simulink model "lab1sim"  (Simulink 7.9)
settings: Solver=ode45  SolverMode=SingleTasking  StartTime=0.0  StopTime=2  FixedStep=0.001  RelTol=1e-3
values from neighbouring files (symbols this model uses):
  C = lC    [initlab1sim.m]
  dDZ = 0.1    [initlab1sim.m]
  dzpos = 0    [initlab1sim.m]
  DZPOS = 0    [initlab1sim.m]
  GAM = lGAM    [initlab1sim.m]
  h = 0.001    [dfa.m]    (also in initlab1sim.m)
  K = lK    [initlab1sim.m]    (also in lqed.m = Phi*Kf+Kv)
  Lc = lLc    (= 1)    [initlab1sim.m]
  Le = lLe    [initlab1sim.m]
  overlap = 0    [fix_opencfg.m]    (also in initlab1sim.m)
  OVERLAP = 2    [initlab1sim.m]
  PHI = lPHI    [initlab1sim.m]
  tl = + 1.3    (= 1.3)    [initlab1sim.m]
  TL = + 1.3    (= 1.3)    [initlab1sim.m]
  tu = - 1.0    (= -1)    [initlab1sim.m]
  TU = - 1.0    (= -1)    [initlab1sim.m]
undefined symbols (not defined in the file or in its folder): DiscIntNeverNeededParam, SimDen, SimNum
libraries: simulink x2, simulink_extras x1

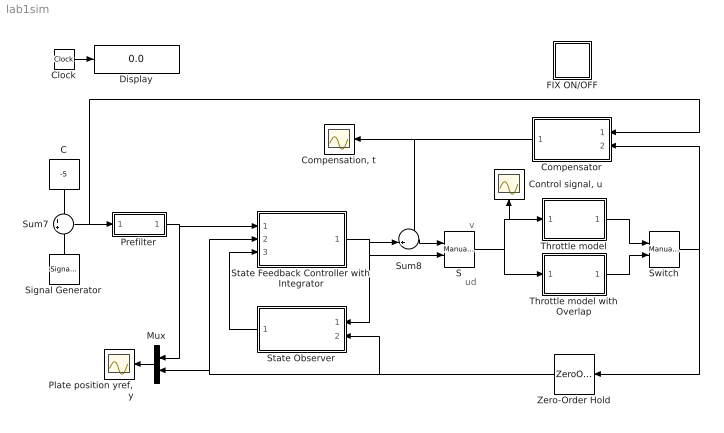
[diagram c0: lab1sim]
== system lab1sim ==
  note: v
  note: ud
  C : Constant  Value=-5
  Clock : Clock
  "Compensation, t" : Scope
  Compensator : Subsystem
  "Control signal, u" : Scope
  Display : Display
  FIX ON/OFF : Subsystem  Description=Fix ON/OFF
  Mux : Mux  Inputs=2
  "Plate position yref, y" : Scope
  Prefilter : Subsystem
  S : simulink/Signal Routing/Manual Switch  sw=0  action=0  varsize=off
  Signal Generator : SignalGenerator  WaveForm=square  Amplitude=5
  State Feedback Controller with Integrator : Subsystem
  State Observer : Subsystem
  Sum7 : Sum
  Sum8 : Sum  Inputs=-+|
  Switch : simulink/Signal Routing/Manual Switch  sw=1  action=0  varsize=off
  Throttle model : Subsystem
  Throttle model with Overlap : Subsystem
  Zero-Order Hold : ZeroOrderHold  SampleTime=h
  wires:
  Signal Generator/1 -> Sum7/2
  Prefilter/1(rfiltered) -> Mux/1, State Feedback Controller with Integrator/1(yr)
  Mux/1 -> "Plate position yref, y"/1
  Zero-Order Hold/1 -> State Observer/2(y), Mux/2, State Feedback Controller with Integrator/2(y)
  State Observer/1(xhat) -> State Feedback Controller with Integrator/3(xhat)
  Sum7/1 -> Prefilter/1(r), Compensator/1(ref.value)
  Switch/1 -> Zero-Order Hold/1, Compensator/2(y)
  Sum8/1 -> S/1
  State Feedback Controller with Integrator/1(ud) -> Sum8/2, S/2, State Observer/1(u)
  Throttle model with Overlap/1(y) -> Switch/2
  Throttle model/1(y) -> Switch/1
  S/1 -> Throttle model/1(u), "Control signal, u"/1, Throttle model with Overlap/1(u)
  Compensator/1(t) -> Sum8/1, "Compensation, t"/1
  Clock/1 -> Display/1
  C/1 -> Sum7/1

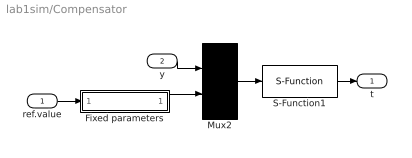
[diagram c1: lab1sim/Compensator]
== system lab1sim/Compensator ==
  ref.value : Inport
  y : Inport  Port=2
  Fixed parameters : Subsystem
  Mux2 : Mux  Inputs=2
  S-Function1 : S-Function  FunctionName=compensator2  Parameters=h overlap/2 -overlap/2  EnableBusSupport=off
  t : Outport
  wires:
  ref.value/1 -> Fixed parameters/1(ref value)
  y/1 -> Mux2/1
  Mux2/1 -> S-Function1/1
  S-Function1/1 -> t/1
  Fixed parameters/1(params) -> Mux2/2

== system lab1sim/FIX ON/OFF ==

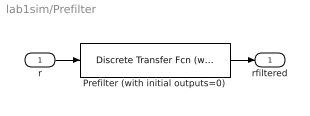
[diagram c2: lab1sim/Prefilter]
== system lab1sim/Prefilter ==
  r : Inport
  Prefilter (with initial outputs=0) : simulink_extras/Additional Discrete/Discrete Transfer Fcn (with initial outputs)  N=[21.3 1 -20.3]  D=[835 -1596 763]  U0=[0]  Y0=0  TS=h
  rfiltered : Outport
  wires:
  Prefilter (with initial outputs=0)/1 -> rfiltered/1
  r/1 -> Prefilter (with initial outputs=0)/1

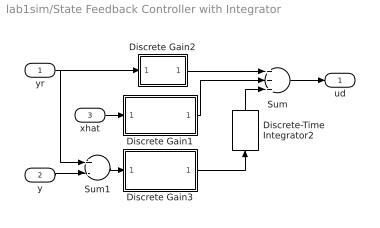
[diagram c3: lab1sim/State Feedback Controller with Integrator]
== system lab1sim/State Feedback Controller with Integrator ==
  yr : Inport
  y : Inport  Port=2
  xhat : Inport  Port=3
  Discrete Gain1 : Subsystem  mask(Discrete Gain){h=h, K=-Le(1:3)}
      mask prompts: h "Sample Time"; K "Gain"
      mask init:
      | s = get_param(gcb,'MaskValueString');
      | s = s(findstr(s,'|')+1:end);
  Discrete Gain2 : Subsystem  mask(Discrete Gain){h=h, K=Lc}
      mask prompts: h "Sample Time"; K "Gain"
      mask init:
      | s = get_param(gcb,'MaskValueString');
      | s = s(findstr(s,'|')+1:end);
  Discrete Gain3 : Subsystem  mask(Discrete Gain){h=h, K=-Le(4)}
      mask prompts: h "Sample Time"; K "Gain"
      mask init:
      | s = get_param(gcb,'MaskValueString');
      | s = s(findstr(s,'|')+1:end);
  Discrete-Time Integrator2 : DiscreteIntegrator  SampleTime=h  ICPrevOutput=DiscIntNeverNeededParam  ICPrevScaledInput=DiscIntNeverNeededParam
  Sum : Sum  Inputs=+++
  Sum1 : Sum  Inputs=+-
  ud : Outport
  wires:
  Discrete Gain1/1(Out1) -> Sum/2
  Discrete-Time Integrator2/1 -> Sum/3
  Sum/1 -> ud/1
  Discrete Gain3/1(Out1) -> Discrete-Time Integrator2/1
  Discrete Gain2/1(Out1) -> Sum/1
  xhat/1 -> Discrete Gain1/1(In1)
  y/1 -> Sum1/2
  yr/1 -> Discrete Gain2/1(In1), Sum1/1
  Sum1/1 -> Discrete Gain3/1(In1)

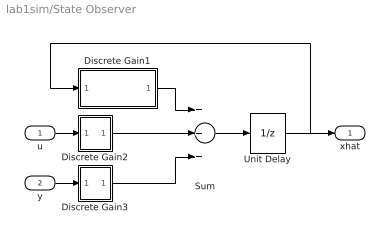
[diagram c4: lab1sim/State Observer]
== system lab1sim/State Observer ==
  u : Inport
  y : Inport  Port=2
  Discrete Gain1 : Subsystem  mask(Discrete Gain){h=h, K=PHI-K*C}
      mask prompts: h "Sample Time"; K "Gain"
      mask init:
      | s = get_param(gcb,'MaskValueString');
      | s = s(findstr(s,'|')+1:end);
  Discrete Gain2 : Subsystem  mask(Discrete Gain){h=h, K=GAM}
      mask prompts: h "Sample Time"; K "Gain"
      mask init:
      | s = get_param(gcb,'MaskValueString');
      | s = s(findstr(s,'|')+1:end);
  Discrete Gain3 : Subsystem  mask(Discrete Gain){h=h, K=K}
      mask prompts: h "Sample Time"; K "Gain"
      mask init:
      | s = get_param(gcb,'MaskValueString');
      | s = s(findstr(s,'|')+1:end);
  Sum : Sum  Inputs=+++
  Unit Delay : UnitDelay  SampleTime=h
  xhat : Outport
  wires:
  Discrete Gain1/1(Out1) -> Sum/1
  Discrete Gain2/1(Out1) -> Sum/2
  Discrete Gain3/1(Out1) -> Sum/3
  Sum/1 -> Unit Delay/1
  Unit Delay/1 -> Discrete Gain1/1(In1), xhat/1
  u/1 -> Discrete Gain2/1(In1)
  y/1 -> Discrete Gain3/1(In1)

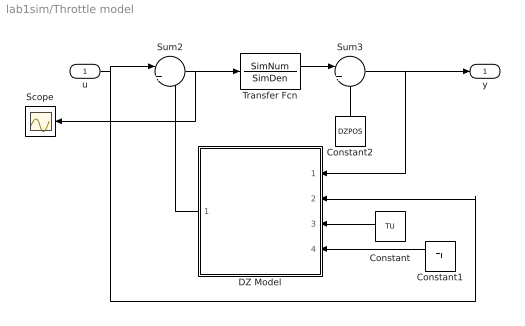
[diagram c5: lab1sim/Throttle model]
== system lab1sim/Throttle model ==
  u : Inport
  Constant : Constant  Value=TU
  Constant1 : Constant  Value=TL
  Constant2 : Constant  Value=DZPOS
  DZ Model : Subsystem
  Scope : Scope
  Sum2 : Sum  Inputs=|++
  Sum3 : Sum  Inputs=|++
  Transfer Fcn : TransferFcn  Numerator=SimNum  Denominator=SimDen
  y : Outport
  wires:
  Sum3/1 -> DZ Model/1(position), y/1
  Constant2/1 -> Sum3/2
  Transfer Fcn/1 -> Sum3/1
  u/1 -> DZ Model/2(torque), Sum2/1
  Constant/1 -> DZ Model/3(TU)
  Constant1/1 -> DZ Model/4(TL)
  Sum2/1 -> Transfer Fcn/1, Scope/1
  DZ Model/1(dz) -> Sum2/2

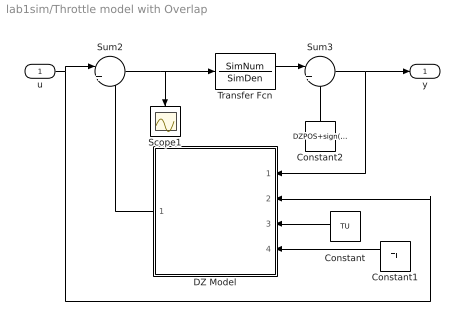
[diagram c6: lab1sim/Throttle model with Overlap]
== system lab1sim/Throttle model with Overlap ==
  u : Inport
  Constant : Constant  Value=TU
  Constant1 : Constant  Value=TL
  Constant2 : Constant  Value=DZPOS+sign(TU+TL)*OVERLAP/2
  DZ Model : Subsystem
  Scope1 : Scope
  Sum2 : Sum  Inputs=|++
  Sum3 : Sum  Inputs=|++
  Transfer Fcn : TransferFcn  Numerator=SimNum  Denominator=SimDen
  y : Outport
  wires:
  Sum3/1 -> DZ Model/1(position), y/1
  Constant2/1 -> Sum3/2
  Transfer Fcn/1 -> Sum3/1
  Sum2/1 -> Scope1/1, Transfer Fcn/1
  Constant1/1 -> DZ Model/4(TL)
  Constant/1 -> DZ Model/3(TU)
  u/1 -> DZ Model/2(torque), Sum2/1
  DZ Model/1(dz) -> Sum2/2

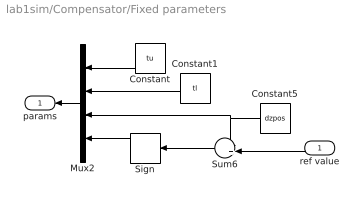
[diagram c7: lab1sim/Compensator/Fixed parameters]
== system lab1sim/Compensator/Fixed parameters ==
  ref value : Inport
  Constant : Constant  Value=tu
  Constant1 : Constant  Value=tl
  Constant5 : Constant  Value=dzpos
  Mux2 : Mux
  Sign : Signum
  Sum6 : Sum  Inputs=-+|
  params : Outport
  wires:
  Sign/1 -> Mux2/4
  Constant/1 -> Mux2/1
  Constant5/1 -> Mux2/3, Sum6/1
  ref value/1 -> Sum6/2
  Sum6/1 -> Sign/1
  Constant1/1 -> Mux2/2
  Mux2/1 -> params/1

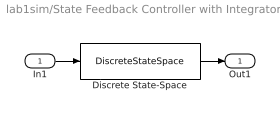
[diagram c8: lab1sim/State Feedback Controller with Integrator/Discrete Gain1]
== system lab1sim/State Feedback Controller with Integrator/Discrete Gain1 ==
  In1 : Inport
  Discrete State-Space : DiscreteStateSpace  A=0  B=zeros(1,size(K,2))  C=zeros(size(K,1),1)  D=K  SampleTime=h
  Out1 : Outport
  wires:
  Discrete State-Space/1 -> Out1/1
  In1/1 -> Discrete State-Space/1

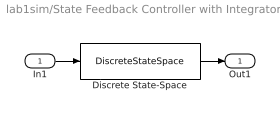
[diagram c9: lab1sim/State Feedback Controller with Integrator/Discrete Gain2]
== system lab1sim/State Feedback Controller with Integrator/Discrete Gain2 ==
  In1 : Inport
  Discrete State-Space : DiscreteStateSpace  A=0  B=zeros(1,size(K,2))  C=zeros(size(K,1),1)  D=K  SampleTime=h
  Out1 : Outport
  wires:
  Discrete State-Space/1 -> Out1/1
  In1/1 -> Discrete State-Space/1

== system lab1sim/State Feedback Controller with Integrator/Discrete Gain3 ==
  In1 : Inport
  Discrete State-Space : DiscreteStateSpace  A=0  B=zeros(1,size(K,2))  C=zeros(size(K,1),1)  D=K  SampleTime=h
  Out1 : Outport
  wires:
  In1/1 -> Discrete State-Space/1
  Discrete State-Space/1 -> Out1/1

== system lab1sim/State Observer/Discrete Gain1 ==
  In1 : Inport
  Discrete State-Space : DiscreteStateSpace  A=0  B=zeros(1,size(K,2))  C=zeros(size(K,1),1)  D=K  SampleTime=h
  Out1 : Outport
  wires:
  Discrete State-Space/1 -> Out1/1
  In1/1 -> Discrete State-Space/1

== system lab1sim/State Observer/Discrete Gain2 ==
  In1 : Inport
  Discrete State-Space : DiscreteStateSpace  A=0  B=zeros(1,size(K,2))  C=zeros(size(K,1),1)  D=K  SampleTime=h
  Out1 : Outport
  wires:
  In1/1 -> Discrete State-Space/1
  Discrete State-Space/1 -> Out1/1

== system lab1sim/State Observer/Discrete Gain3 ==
  In1 : Inport
  Discrete State-Space : DiscreteStateSpace  A=0  B=zeros(1,size(K,2))  C=zeros(size(K,1),1)  D=K  SampleTime=h
  Out1 : Outport
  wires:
  Discrete State-Space/1 -> Out1/1
  In1/1 -> Discrete State-Space/1

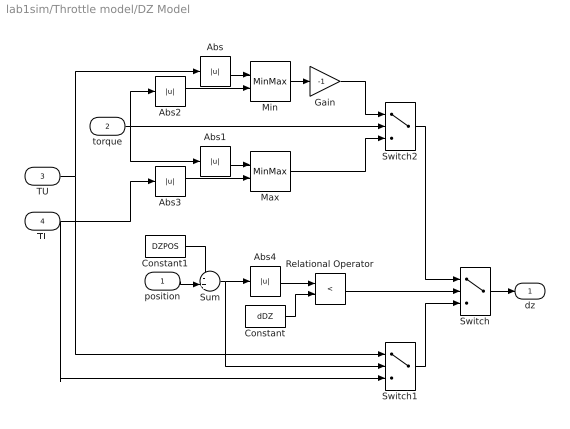
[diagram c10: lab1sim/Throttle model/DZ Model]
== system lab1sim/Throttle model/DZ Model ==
  position : Inport
  torque : Inport  Port=2
  TU : Inport  Port=3
  TL : Inport  Port=4
  Abs{,1..4} (5 alike) : Abs
  Constant : Constant  Value=dDZ
  Constant1 : Constant  Value=DZPOS
  Gain : Gain  Gain=-1
  Max : MinMax  Inputs=2
  Min : MinMax  Inputs=2
  Relational Operator : RelationalOperator  Operator=<
  Sum : Sum  Inputs=-+|
  Switch : Switch  Threshold=0.5
  Switch1 : Switch
  Switch2 : Switch
  dz : Outport  InitialOutput=0
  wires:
  Abs4/1 -> Relational Operator/1
  Relational Operator/1 -> Switch/2
  Max/1 -> Switch2/3
  TL/1 -> Switch1/3, Abs3/1
  torque/1 -> Switch2/2, Abs1/1, Abs2/1
  TU/1 -> Switch1/1, Abs/1
  Abs/1 -> Min/1
  Abs1/1 -> Max/1
  Min/1 -> Gain/1
  Gain/1 -> Switch2/1
  Abs2/1 -> Min/2
  Abs3/1 -> Max/2
  Switch2/1 -> Switch/1
  Switch1/1 -> Switch/3
  Switch/1 -> dz/1
  Constant/1 -> Relational Operator/2
  position/1 -> Sum/2
  Constant1/1 -> Sum/1
  Sum/1 -> Abs4/1, Switch1/2

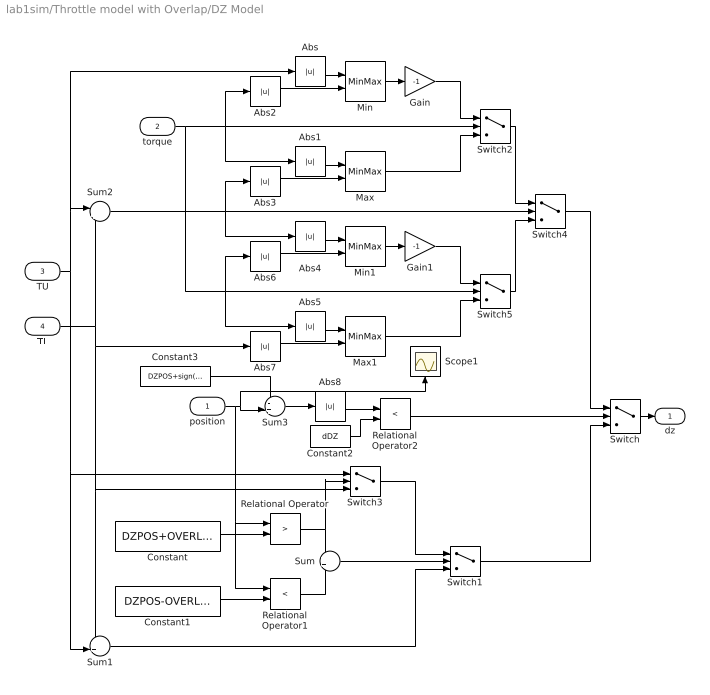
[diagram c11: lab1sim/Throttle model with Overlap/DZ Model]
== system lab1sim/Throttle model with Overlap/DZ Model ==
  position : Inport
  torque : Inport  Port=2
  TU : Inport  Port=3
  TL : Inport  Port=4
  Abs{,1..8} (9 alike) : Abs
  Constant : Constant  Value=DZPOS+OVERLAP/2
  Constant1 : Constant  Value=DZPOS-OVERLAP/2
  Constant2 : Constant  Value=dDZ
  Constant3 : Constant  Value=DZPOS+sign(TU+TL)*OVERLAP/2
  Gain : Gain  Gain=-1
  Gain1 : Gain  Gain=-1
  Max : MinMax  Inputs=2
  Max1 : MinMax  Inputs=2
  Min : MinMax  Inputs=2
  Min1 : MinMax  Inputs=2
  Relational Operator : RelationalOperator  Operator=>
  Relational Operator1 : RelationalOperator  Operator=<
  Relational Operator2 : RelationalOperator  Operator=<
  Scope1 : Scope
  Sum : Sum
  Sum1 : Sum  Inputs=++|
  Sum2 : Sum  Inputs=|++
  Sum3 : Sum  Inputs=-+|
  Switch : Switch  Threshold=0.5
  Switch1 : Switch  Threshold=0.5
  Switch2 : Switch
  Switch3 : Switch  Threshold=0.5
  Switch4 : Switch
  Switch5 : Switch
  dz : Outport  InitialOutput=0
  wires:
  Abs8/1 -> Relational Operator2/1
  Relational Operator2/1 -> Switch/2
  Sum3/1 -> Abs8/1
  Constant2/1 -> Relational Operator2/2
  Constant3/1 -> Sum3/1
  position/1 -> Scope1/1, Sum3/2, Relational Operator/1, Relational Operator1/1
  TL/1 -> Sum2/2, Sum1/1, Switch3/3, Abs7/1
  TU/1 -> Switch3/1, Sum1/2, Sum2/1, Abs/1
  Abs/1 -> Min/1
  Abs1/1 -> Max/1
  Min/1 -> Gain/1
  Gain/1 -> Switch2/1
  Abs2/1 -> Min/2
  Abs3/1 -> Max/2
  Max1/1 -> Switch5/3
  Abs4/1 -> Min1/1
  Abs5/1 -> Max1/1
  Abs6/1 -> Min1/2
  Abs7/1 -> Max1/2
  Constant/1 -> Relational Operator/2
  Constant1/1 -> Relational Operator1/2
  Relational Operator1/1 -> Sum/2
  Sum/1 -> Switch1/2
  Sum1/1 -> Switch1/3
  Switch3/1 -> Switch1/1
  Relational Operator/1 -> Sum/1, Switch3/2
  Switch1/1 -> Switch/3
  torque/1 -> Switch2/2, Abs1/1, Abs2/1, Switch5/2, Abs6/1, Abs5/1
  Switch2/1 -> Switch4/1
  Switch5/1 -> Switch4/3
  Switch/1 -> dz/1
  Switch4/1 -> Switch/1
  Sum2/1 -> Switch4/2, Abs3/1, Abs4/1
  Max/1 -> Switch2/3
  Min1/1 -> Gain1/1
  Gain1/1 -> Switch5/1
